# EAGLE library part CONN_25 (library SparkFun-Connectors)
Multi connection point. Often used as Generic Header-pin footprint for 0.1 inch spaced/style header connections On any of the 0.1 inch spaced packages, you can populate with these: Break Away Headers - Straight (PRT-00116) Break Away Male Headers - Right Angle (PRT-00553) Female Headers (PRT-00115) Break Away Headers - Machine Pin (PRT-00117) Break Away Female Headers - Swiss Machine Pin (PRT-00743) For SCREWTERMINALS and SPRING TERMINALS visit here: Screw Terimnals on SparkFun.com (5mm/3.5mm/2.54mm spacing) This device is also useful as a general connection point to wire up your design to another part of your project. Our various solder wires solder well into these plated through hole pads. Hook-Up Wire - Assortment (Stranded, 22 AWG) (PRT-11375) Hook-Up Wire - Assortment (Solid Core, 22 AWG) (PRT-11367) View the entire wire category on our website here Special notes: Molex polarized connector foot print use with SKU : PRT-08231 with associated crimp pins and housings. 1MM SMD Version SKU: PRT-10208 NOTES ON THE VARIANTS LOCK and LOCK_LONGPADS... This footprint was designed to help hold the alignment of a through-hole component (i.e. 6-pin header) while soldering it into place. You may notice that each hole has been shifted either up or down by 0.005 of an inch from it's more standard position (which is a perfectly straight line). This slight alteration caused the pins (the squares in the middle) to touch the edges of the holes. Because they are alternating, it causes a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
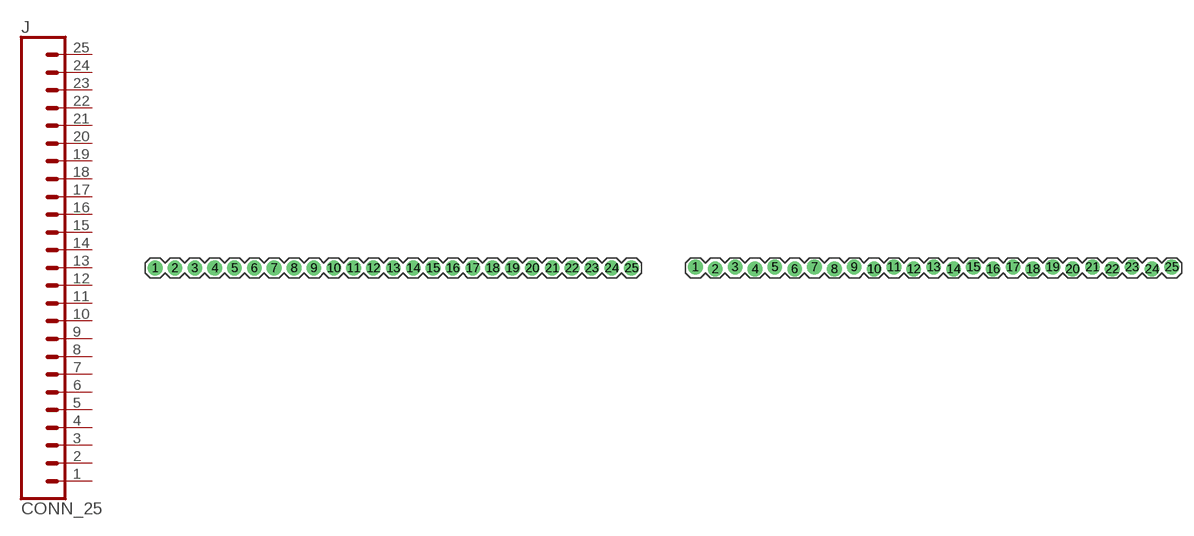
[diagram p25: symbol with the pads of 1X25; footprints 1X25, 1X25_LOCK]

Designator prefix J

## CONN_25  [1X25]
1  1  pas
2  2  pas
3  3  pas
4  4  pas
5  5  pas
6  6  pas
7  7  pas
8  8  pas
9  9  pas
10  10  pas
11  11  pas
12  12  pas
13  13  pas
14  14  pas
15  15  pas
16  16  pas
17  17  pas
18  18  pas
19  19  pas
20  20  pas
21  21  pas
22  22  pas
23  23  pas
24  24  pas
25  25  pas

## CONN_25LOCK  [1X25_LOCK]
Pads as for 1X25

## CONN_25LOCK_LONGPADS  [1X25_LOCK_LONGPADS]
Pads as for 1X25

## CONN_25PTH_LONGPADS  [1X25_LONGPAD]
Pads as for 1X25

## Footprint 1X25 (pad centres in mm)
Plated Through Hole -25 Specifications: Pin count:25 Pin pitch:0.1" Example device(s): CONN_25
drill 1.016 pad 1.88: 1 0,0; 2 2.54,0; 3 5.08,0; 4 7.62,0; 5 10.16,0; 6 12.7,0; 7 15.24,0; 8 17.78,0; 9 20.32,0; 10 22.86,0; 11 25.4,0; 12 27.94,0; 13 30.48,0; 14 33.02,0; 15 35.56,0; 16 38.1,0; 17 40.64,0; 18 43.18,0; 19 45.72,0; 20 48.26,0; 21 50.8,0; 22 53.34,0; 23 55.88,0; 24 58.42,0; 25 60.96,0

## Footprint 1X25_LOCK (pad centres in mm)
Plated Through Hole -25 pin Locking Footprint Holes are offset 0.005" from center, to hold pins in place while soldering. Specifications: Pin count:25 Pin pitch:0.1" Example device(s): CONN_25
drill 1.016 pad 1.88: 1 0,0.127; 2 2.54,-0.127; 3 5.08,0.127; 4 7.62,-0.127; 5 10.16,0.127; 6 12.7,-0.127; 7 15.24,0.127; 8 17.78,-0.127; 9 20.32,0.127; 10 22.86,-0.127; 11 25.4,0.127; 12 27.94,-0.127; 13 30.48,0.127; 14 33.02,-0.127; 15 35.56,0.127; 16 38.1,-0.127; 17 40.64,0.127; 18 43.18,-0.127; 19 45.72,0.127; 20 48.26,-0.127; 21 50.8,0.127; 22 53.34,-0.127; 23 55.88,0.127; 24 58.42,-0.127; 25 60.96,0.127

## Footprint 1X25_LOCK_LONGPADS (pad centres in mm)
Plated Through Hole -25 pin Locking Footprint w/ Long Pads Holes are offset 0.005" from center, to hold pins in place while soldering. Specifications: Pin count:25 Pin pitch:0.1" Example device(s):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
drill 1.016 long: 1 0,0.127; 2 2.54,-0.127; 3 5.08,0.127; 4 7.62,-0.127; 5 10.16,0.127; 6 12.7,-0.127; 7 15.24,0.127; 8 17.78,-0.127; 9 20.32,0.127; 10 22.86,-0.127; 11 25.4,0.127; 12 27.94,-0.127; 13 30.48,0.127; 14 33.02,-0.127; 15 35.56,0.127; 16 38.1,-0.127; 17 40.64,0.127; 18 43.18,-0.127; 19 45.72,0.127; 20 48.26,-0.127; 21 50.8,0.127; 22 53.34,-0.127; 23 55.88,0.127; 24 58.42,-0.127; 25 60.96,0.127

## Footprint 1X25_LONGPAD (pad centres in mm)
Plated Through Hole -25 pin Long Pads Specifications: Pin count:25 Pin pitch:0.1" Example device(s): CONN_25
drill 1.118 long: 1 0,0; 2 2.54,0; 3 5.08,0; 4 7.62,0; 5 10.16,0; 6 12.7,0; 7 15.24,0; 8 17.78,0; 9 20.32,0; 10 22.86,0; 11 25.4,0; 12 27.94,0; 13 30.48,0; 14 33.02,0; 15 35.56,0; 16 38.1,0; 17 40.64,0; 18 43.18,0; 19 45.72,0; 20 48.26,0; 21 50.8,0; 22 53.34,0; 23 55.88,0; 24 58.42,0; 25 60.96,0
